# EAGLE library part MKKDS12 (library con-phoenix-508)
PHOENIX
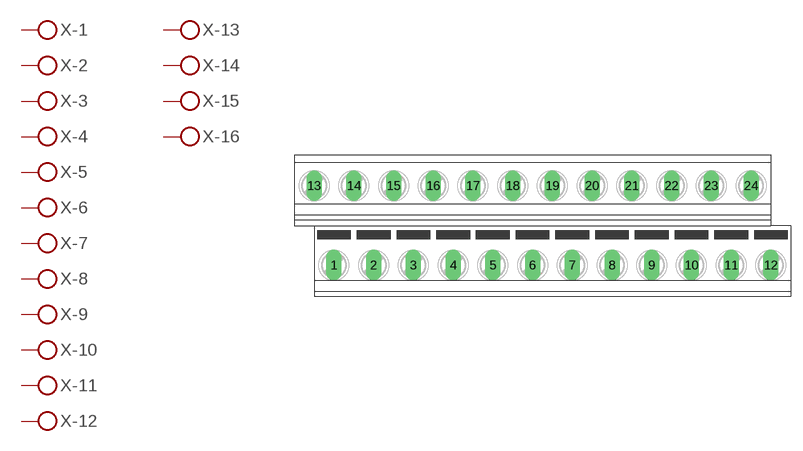
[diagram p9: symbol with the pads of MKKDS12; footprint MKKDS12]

Designator prefix X; gates -1=KL -2=KL -3=KL -4=KL -5=KL -6=KL -7=KL -8=KL -9=KL -10=KL -11=KL -12=KL -13=KL -14=KL -15=KL -16=KL -17=KL -18=KL -19=KL -20=KL -21=KL -22=KL -23=KL -24=KLV

## MKKDS12 (OC_FARNELL: unknown; OC_NEWARK: unknown)  [MKKDS12]
1  -1:KL  pas
2  -2:KL  pas
3  -3:KL  pas
4  -4:KL  pas
5  -5:KL  pas
6  -6:KL  pas
7  -7:KL  pas
8  -8:KL  pas
9  -9:KL  pas
10  -10:KL  pas
11  -11:KL  pas
12  -12:KL  pas
13  -13:KL  pas
14  -14:KL  pas
15  -15:KL  pas
16  -16:KL  pas
17  -17:KL  pas
18  -18:KL  pas
19  -19:KL  pas
20  -20:KL  pas
21  -21:KL  pas
22  -22:KL  pas
23  -23:KL  pas
24  -24:KL  pas

## Footprint MKKDS12 (pad centres in mm)
PHOENIX MKKDSN 1,5/ 8-5,08 Source: http://eshop.phoenixcontact.com .. 1726202.pdf
drill 1.321 long: 1 -26.67,-4.445; 2 -21.59,-4.445; 3 -16.51,-4.445; 4 -11.43,-4.445; 5 -6.35,-4.445; 6 -1.27,-4.445; 7 3.81,-4.445; 8 8.89,-4.445; 9 13.97,-4.445; 10 19.05,-4.445; 11 24.13,-4.445; 12 29.21,-4.445; 13 -29.21,5.715; 14 -24.13,5.715; 15 -19.05,5.715; 16 -13.97,5.715; 17 -8.89,5.715; 18 -3.81,5.715; 19 1.27,5.715; 20 6.35,5.715; 21 11.43,5.715; 22 16.51,5.715; 23 21.59,5.715; 24 26.67,5.715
